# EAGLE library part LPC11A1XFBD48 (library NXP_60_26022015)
32-bit ARM Cortex-M0 microcontroller; up to 32 kB flash, 8 kB SRAM, 4 kB EEPROM; configurable analog/mixed-signal The LPC11Axx are an ARM Cortex-M0 based, low-cost 32-bit MCU family, designed for 8/16-bit microcontroller applications, offering performance, low power, simple instruction set and memory addressing together with reduced code size compared to existing 8/16-bit architectures. The LPC11Axx operate at CPU frequencies of up to 50 MHz. Analog/mixed-signal subsystems can be configured by software from interconnected digital and analog peripherals. The digital peripherals on the LPC11Axx include up to 32 kB of flash memory, up to 4 kB of EEPROM data memory, up to 8 kB of SRAM data memory, a Fast-mode Plus I 2 C-bus interface, a RS-485/EIA-485 USART, two SSP controllers, four general purpose counter/timers, and up to 42 general purpose I/O pins. Analog peripherals include a 10-bit ADC, a 10-bit DAC, an analog comparator, a temperature sensor, an internal voltage reference, and UnderVoltage LockOut (UVLO) protection. AAL Eindhoven MK
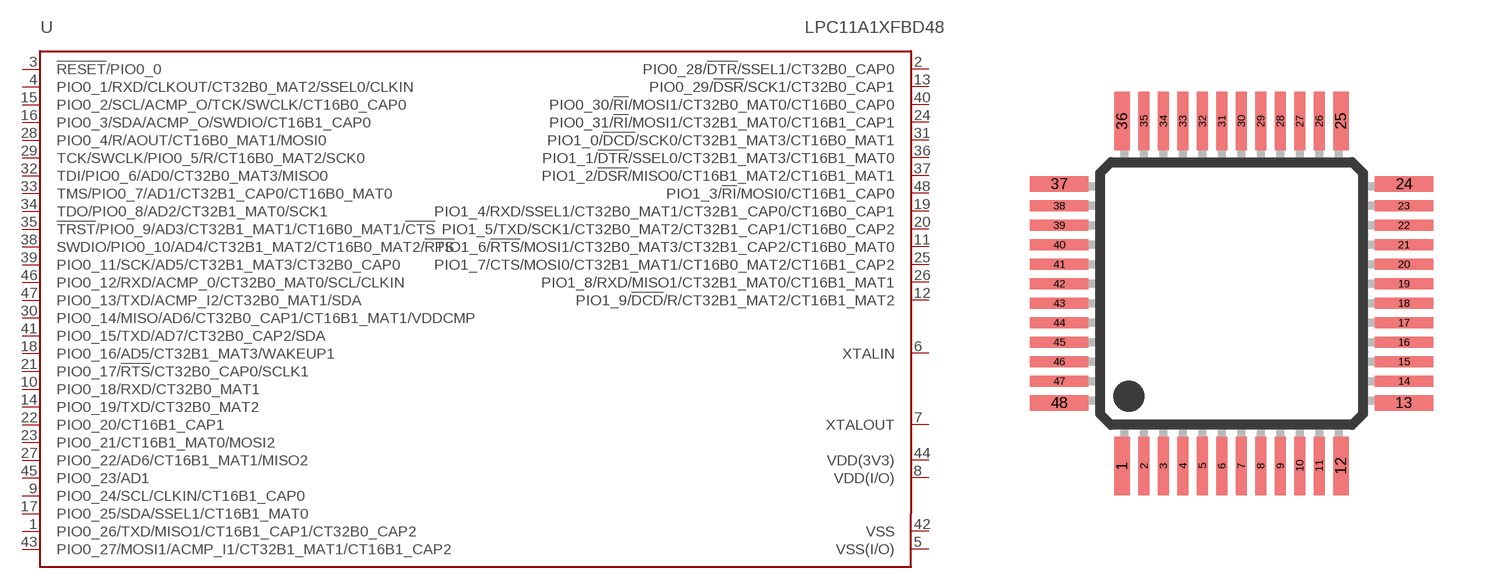
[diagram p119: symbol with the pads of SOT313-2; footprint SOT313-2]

Designator prefix U

## LPC11A1XFBD48  [SOT313-2]
1  PIO0_26/TXD/MISO1/CT16B1_CAP1/CT32B0_CAP2
2  PIO0_28/!DTR!/SSEL1/CT32B0_CAP0
3  !RESET!/PIO0_0
4  PIO0_1/RXD/CLKOUT/CT32B0_MAT2/SSEL0/CLKIN
5  VSS(I/O)  pwr
6  XTALIN  pas
7  XTALOUT  pas
8  VDD(I/O)  pwr
9  PIO0_24/SCL/CLKIN/CT16B1_CAP0
10  PIO0_18/RXD/CT32B0_MAT1
11  PIO1_6/!RTS!/MOSI1/CT32B0_MAT3/CT32B1_CAP2/CT16B0_MAT0
12  PIO1_9/!DCD!/R/CT32B1_MAT2/CT16B1_MAT2
13  PIO0_29/!DSR!/SCK1/CT32B0_CAP1
14  PIO0_19/TXD/CT32B0_MAT2
15  PIO0_2/SCL/ACMP_O/TCK/SWCLK/CT16B0_CAP0
16  PIO0_3/SDA/ACMP_O/SWDIO/CT16B1_CAP0
17  PIO0_25/SDA/SSEL1/CT16B1_MAT0
18  PIO0_16/AD5/CT32B1_MAT3/WAKEUP1
19  PIO1_4/RXD/SSEL1/CT32B0_MAT1/CT32B1_CAP0/CT16B0_CAP1
20  PIO1_5/TXD/SCK1/CT32B0_MAT2/CT32B1_CAP1/CT16B0_CAP2
21  PIO0_17/!RTS!/CT32B0_CAP0/SCLK1
22  PIO0_20/CT16B1_CAP1
23  PIO0_21/CT16B1_MAT0/MOSI2
24  PIO0_31/!RI!/MOSI1/CT32B1_MAT0/CT16B1_CAP1
25  PIO1_7/CTS/MOSI0/CT32B1_MAT1/CT16B0_MAT2/CT16B1_CAP2
26  PIO1_8/RXD/MISO1/CT32B1_MAT0/CT16B1_MAT1
27  PIO0_22/AD6/CT16B1_MAT1/MISO2
28  PIO0_4/R/AOUT/CT16B0_MAT1/MOSI0
29  TCK/SWCLK/PIO0_5/R/CT16B0_MAT2/SCK0
30  PIO0_14/MISO/AD6/CT32B0_CAP1/CT16B1_MAT1/VDDCMP
31  PIO1_0/!DCD!/SCK0/CT32B1_MAT3/CT16B0_MAT1
32  TDI/PIO0_6/AD0/CT32B0_MAT3/MISO0
33  TMS/PIO0_7/AD1/CT32B1_CAP0/CT16B0_MAT0
34  TDO/PIO0_8/AD2/CT32B1_MAT0/SCK1
35  !TRST!/PIO0_9/AD3/CT32B1_MAT1/CT16B0_MAT1/!CTS!
36  PIO1_1/!DTR!/SSEL0/CT32B1_MAT3/CT16B1_MAT0
37  PIO1_2/!DSR!/MISO0/CT16B1_MAT2/CT16B1_MAT1
38  SWDIO/PIO0_10/AD4/CT32B1_MAT2/CT16B0_MAT2/!RTS!
39  PIO0_11/SCK/AD5/CT32B1_MAT3/CT32B0_CAP0
40  PIO0_30/!RI!/MOSI1/CT32B0_MAT0/CT16B0_CAP0
41  PIO0_15/TXD/AD7/CT32B0_CAP2/SDA
42  VSS  pwr
43  PIO0_27/MOSI1/ACMP_I1/CT32B1_MAT1/CT16B1_CAP2
44  VDD(3V3)  pwr
45  PIO0_23/AD1
46  PIO0_12/RXD/ACMP_0/CT32B0_MAT0/SCL/CLKIN
47  PIO0_13/TXD/ACMP_I2/CT32B0_MAT1/SDA
48  PIO1_3/!RI!/MOSI0/CT16B1_CAP0

## Footprint SOT313-2 (pad centres in mm)
SOT313-2 LQFP48: plastic low profile quad flat package; 48 leads; body 7 x 7 x 1.4 mm JEDEC: MS-026 IEC: 136E05 Footprint according to NXP SOT313-2 specification, however the cornerpins are 0.4mm in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
smd 0.4 x 1.5: 1 -2.81,-4.425; 12 2.81,-4.425; 25 2.81,4.425; 36 -2.81,4.425
smd 0.28 x 1.5: 2 -2.25,-4.425; 3 -1.75,-4.425; 4 -1.25,-4.425; 5 -0.75,-4.425; 6 -0.25,-4.425; 7 0.25,-4.425; 8 0.75,-4.425; 9 1.25,-4.425; 10 1.75,-4.425; 11 2.25,-4.425; 26 2.25,4.425; 27 1.75,4.425; 28 1.25,4.425; 29 0.75,4.425; 30 0.25,4.425; 31 -0.25,4.425; 32 -0.75,4.425; 33 -1.25,4.425; 34 -1.75,4.425; 35 -2.25,4.425
smd 1.5 x 0.4: 13 4.425,-2.81; 24 4.425,2.81; 37 -4.425,2.81; 48 -4.425,-2.81
smd 1.5 x 0.28: 14 4.425,-2.25; 15 4.425,-1.75; 16 4.425,-1.25; 17 4.425,-0.75; 18 4.425,-0.25; 19 4.425,0.25; 20 4.425,0.75; 21 4.425,1.25; 22 4.425,1.75; 23 4.425,2.25; 38 -4.425,2.25; 39 -4.425,1.75; 40 -4.425,1.25; 41 -4.425,0.75; 42 -4.425,0.25; 43 -4.425,-0.25; 44 -4.425,-0.75; 45 -4.425,-1.25; 46 -4.425,-1.75; 47 -4.425,-2.25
